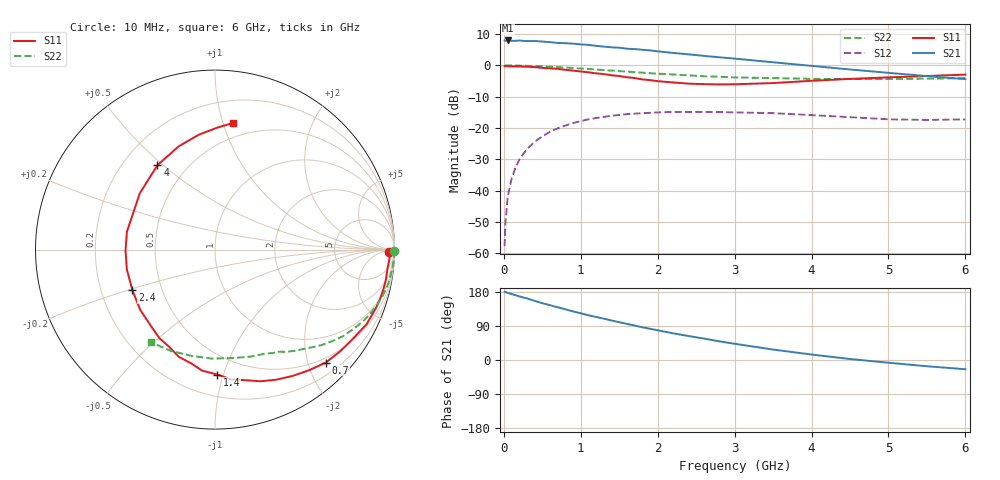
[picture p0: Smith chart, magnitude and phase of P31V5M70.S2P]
! SIEMENS Small Signal Semiconductors
! BFP181
! Si NPN RF Bipolar Junction Transistor in SOT143
! VCE = 1.5 V  IC = 0.7 mA
! Common Emitter S-Parameters:  March  1996
# GHz  S  MA  R  50
!  f  S11  S21  S12  S22
! GHz  MAG  ANG  MAG  ANG  MAG  ANG  MAG  ANG
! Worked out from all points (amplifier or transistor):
!   36 points, 10 MHz to 6 GHz, reference 50 ohm
!   highest |S21| = 8.0 dB at 50 MHz (marker M1)
!   |S21| within 3 dB of that: start of sweep to 1.816 GHz
!   unconditionally stable (mu >= 1): 3.413 GHz to end of sweep
!   at 250 MHz: K = 0.08, MSG = 18.1 dB, |S12| = -28.3 dB
!   at 1.4 GHz: K = 0.47, MSG = 10.9 dB, |S12| = -16.1 dB
!   at 6 GHz: K = 1.39, MAG = 2.7 dB, |S12| = -17.2 dB
!   S11 on the Smith chart (normalised r, x): 10 MHz: 57, -28; 700 MHz: 0.41, -2.32; 1.4 GHz: 0.35, -0.95; 2.4 GHz: 0.34, -0.21; 4 GHz: 0.34, +0.48; 6 GHz: 0.38, +1.08
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0.01  0.9722 -0.8  2.503 179.8  0.0013 84.9  0.9998 -0.3
0.02  0.9754 -1.2  2.482 179.5  0.003 92.1  0.9975 -0.7
0.05  0.9731 -3.1  2.508 177.0  0.0079 89.5  0.9974 -1.6
0.1  0.9665 -6.6  2.481 174.2  0.0154 85.1  0.9991 -3.2
0.15  0.9668 -10.1  2.471 171.0  0.0231 82.0  0.9946 -4.7
0.2  0.964 -13.2  2.503 168.0  0.031 80.8  0.9932 -6.4
0.25  0.9599 -16.8  2.469 165.0  0.0383 78.6  0.9893 -8.0
0.4  0.9412 -26.3  2.458 156.0  0.0604 72.0  0.9795 -12.5
0.5  0.9147 -33.0  2.409 150.0  0.0737 67.4  0.9683 -15.6
0.7  0.882 -45.5  2.29 139.1  0.099 59.0  0.9411 -21.3
0.9  0.8266 -58.3  2.233 128.2  0.1204 50.9  0.9106 -26.6
1.1  0.7765 -70.9  2.132 118.0  0.138 43.6  0.8778 -31.4
1.4  0.6962 -88.9  1.948 104.3  0.1571 33.7  0.8284 -38.1
1.8  0.5989 -115.1  1.782 86.3  0.173 23.2  0.7666 -45.2
2.2  0.5351 -141.2  1.585 70.4  0.1808 13.7  0.7175 -51.8
2.4  0.5126 -154.0  1.505 63.3  0.1814 9.5  0.6946 -55.1
3  0.5008 168.6  1.287 42.8  0.178 -0.8  0.6442 -64.1
3.5  0.5234 143.2  1.124 27.6  0.1731 -6.8  0.6279 -71.9
4  0.569 124.3  0.985 14.4  0.1609 -11.1  0.6113 -81.3
4.5  0.6097 109.4  0.863 2.6  0.1494 -13.7  0.6076 -91.8
5.5  0.6788 89.1  0.676 -16.5  0.135 -10.2  0.6154 -113.5
6  0.7134 81.8  0.605 -24.4  0.1376 -7.3  0.6274 -124.7
